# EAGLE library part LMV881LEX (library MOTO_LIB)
LOW NOISE OPAMP with Shutdown.
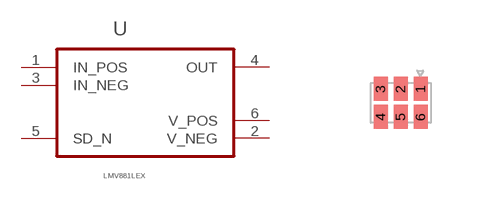
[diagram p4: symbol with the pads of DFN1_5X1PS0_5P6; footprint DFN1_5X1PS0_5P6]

Designator prefix U

## LMV881LEX (MPN: LMV881LEX; SUPPLIER: TI)  [DFN1_5X1PS0_5P6]
1  IN_POS  in
2  V_NEG  pwr
3  IN_NEG  in
4  OUT  out
5  SD_N  in
6  V_POS  pwr

## Footprint DFN1_5X1PS0_5P6 (pad centres in mm)
smd 0.35 x 0.6: 1 0.5,0.35; 2 0,0.35; 3 -0.5,0.35; 4 -0.5,-0.35; 5 0,-0.35; 6 0.5,-0.35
